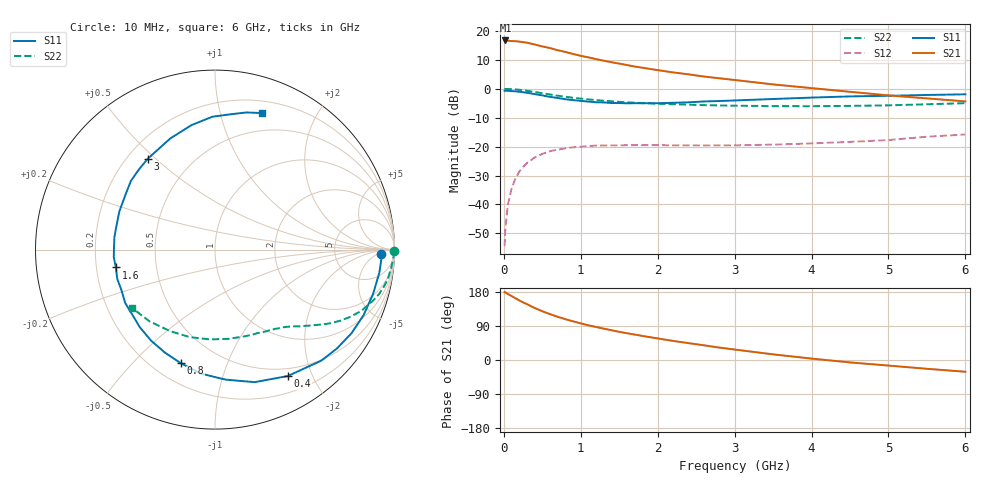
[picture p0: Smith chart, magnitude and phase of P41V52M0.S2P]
! SIEMENS Small Signal Semiconductors
! BFP182
! Si NPN RF Bipolar Junction Transistor in SOT143
! VCE = 1.5 V  IC = 2 mA
! Common Emitter S-Parameters:  March  1996
# GHz  S  MA  R  50
!  f  S11  S21  S12  S22
! GHz  MAG  ANG  MAG  ANG  MAG  ANG  MAG  ANG
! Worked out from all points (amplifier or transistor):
!   36 points, 10 MHz to 6 GHz, reference 50 ohm
!   highest |S21| = 16.7 dB at 20 MHz (marker M1)
!   |S21| within 3 dB of that: start of sweep to 650.1 MHz
!   unconditionally stable (mu >= 1): 2.137 GHz to end of sweep
!   at 250 MHz: K = 0.13, MSG = 21.6 dB, |S12| = -27.0 dB
!   at 1.4 GHz: K = 0.69, MSG = 14.4 dB, |S12| = -19.6 dB
!   at 6 GHz: K = 1.01, MAG = 5.2 dB, |S12| = -15.8 dB
!   S11 on the Smith chart (normalised r, x): 10 MHz: 23, -8; 400 MHz: 0.40, -1.66; 800 MHz: 0.31, -0.70; 1.6 GHz: 0.28, -0.08; 3 GHz: 0.28, +0.47; 6 GHz: 0.31, +1.36
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0.01  0.9251 -1.6  6.808 179.2  0.0019 86.3  0.9955 -0.6
0.02  0.9285 -3.1  6.874 178.4  0.0039 84.3  0.997 -1.3
0.05  0.9247 -8.0  6.82 174.4  0.0095 87.5  0.9936 -3.2
0.1  0.9147 -15.7  6.72 168.8  0.0187 79.6  0.9855 -6.4
0.2  0.8919 -31.5  6.57 157.4  0.0369 72.0  0.9634 -12.4
0.3  0.8563 -46.3  6.293 147.5  0.0521 63.2  0.9253 -17.9
0.4  0.8126 -60.1  5.863 137.3  0.0649 56.1  0.8841 -22.7
0.5  0.771 -73.3  5.417 128.7  0.075 49.6  0.8409 -26.5
0.6  0.727 -85.3  5.082 121.0  0.0835 44.0  0.7996 -29.8
0.7  0.6953 -96.4  4.661 114.1  0.0887 39.3  0.762 -32.6
0.8  0.6615 -106.6  4.349 107.6  0.0934 35.2  0.7288 -34.9
1  0.62 -124.9  3.722 96.6  0.0999 28.4  0.6782 -38.6
1.1  0.6023 -134.0  3.504 91.5  0.1026 25.9  0.657 -40.3
1.3  0.5821 -149.3  3.065 82.7  0.105 21.1  0.6227 -43.3
1.6  0.5614 -169.8  2.583 70.7  0.1063 16.8  0.5851 -47.4
1.8  0.5628 178.3  2.323 63.5  0.1065 15.0  0.5689 -50.1
2.2  0.5739 158.2  1.925 50.4  0.1054 12.2  0.542 -56.2
3  0.63 126.4  1.424 27.6  0.1055 11.5  0.5111 -70.8
3.5  0.6675 111.9  1.194 14.9  0.1084 12.4  0.5029 -81.3
4.5  0.7404 91.2  0.889 -6.4  0.1211 14.7  0.5075 -106.1
5.5  0.7838 77.1  0.684 -23.2  0.1487 15.2  0.5413 -132.4
6  0.805 70.9  0.607 -31.0  0.1623 12.3  0.5653 -145.0
